(* Logix 5000 AddOnInstructionDefinition export; software revision 16.04 *)

ADD_ON_INSTRUCTION AMCI_ANG1E_Absolute_Move   (* revision 1.1, vendor AMCI *)
// Revision note:
// Version 1.1 added the slot_axis number and the input parameters can now be tags or discrete values.
VAR_INPUT
   slot_axis_number : INT; {required}
   Target_Position : DINT; {required}
   Programmed_Speed : DINT; {required}
   Acceleration : INT; {required}
   Deceleration : INT; {required}
END_VAR
VAR_IN_OUT
   AMCI_ANG1E_output_data : INT[10]; {required}
END_VAR
VAR
   Upper_Result_X_1000 : DINT;
   command_data_block : INT[10];
        [0]   // Command Bits MSW
        [1]   // Command Bits LSW
        [2]   // Upper Target Position
        [3]   // Lower Target Position
        [4]   // Upper Programmed Speed
        [5]   // Lower Programmed Speed
   index : INT;
END_VAR

ROUTINE Logic   (* ladder *)
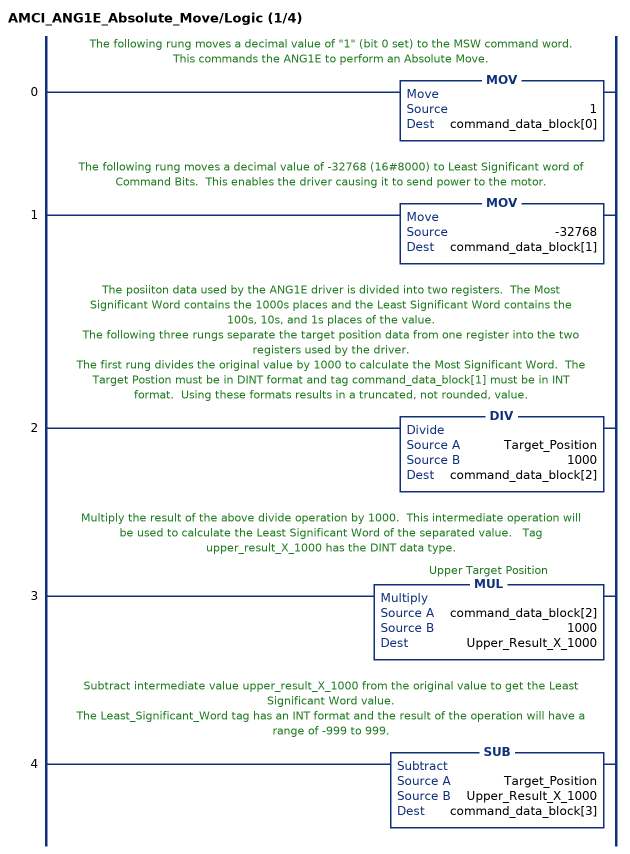
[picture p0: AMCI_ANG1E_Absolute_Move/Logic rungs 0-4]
   // The following rung moves a decimal value of "1" (bit 0 set) to the MSW command word.  This commands the ANG1E to perform an Absolute Move.
   0: MOV(1,command_data_block[0]);
   // The following rung moves a decimal value of -32768 (16#8000) to Least Significant word of Command Bits.  This enables the driver causing it to send power to the motor.
   1: MOV(-32768,command_data_block[1]);
   // The posiiton data used by the ANG1E driver is divided into two registers.  The Most Significant Word contains the 1000s places and the Least Significant Word contains the 100s, 10s, and 1s places of the value.
   // The following three rungs separate the target position data from one register into the two registers used by the driver.
   // The first rung divides the original value by 1000 to calculate the Most Significant Word.  The Target Postion must be in DINT format and tag command_data_block[1] must be in INT format.  Using these formats results in a truncated, not rounded, value.
   2: DIV(Target_Position,1000,command_data_block[2]);
   // Multiply the result of the above divide operation by 1000.  This intermediate operation will be used to calculate the Least Significant Word of the separated value.   Tag upper_result_X_1000 has the DINT data type.
   3: MUL(command_data_block[2],1000,Upper_Result_X_1000);
   // Subtract intermediate value upper_result_X_1000 from the original value to get the Least Significant Word value.
   // The Least_Significant_Word tag has an INT format and the result of the operation will have a range of -999 to 999.
   4: SUB(Target_Position,Upper_Result_X_1000,command_data_block[3]);
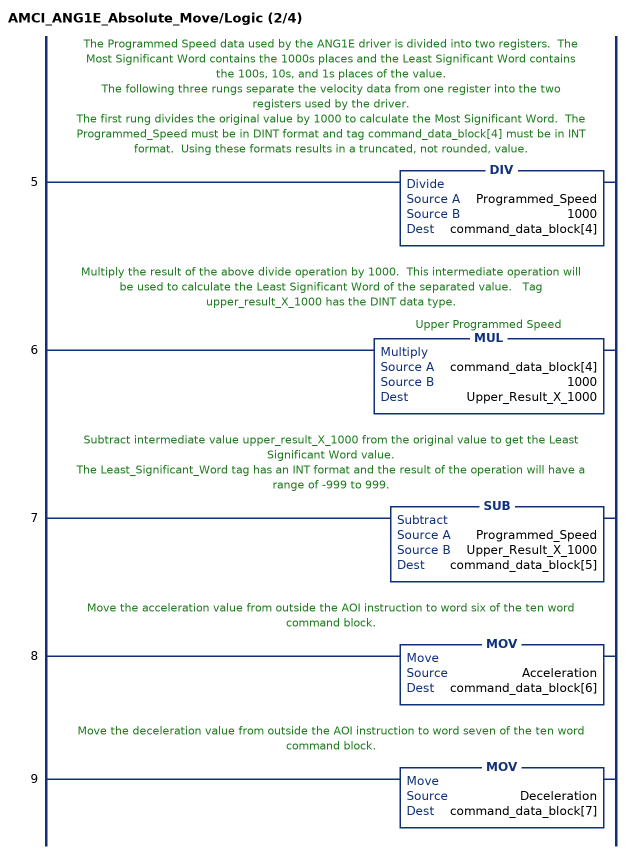
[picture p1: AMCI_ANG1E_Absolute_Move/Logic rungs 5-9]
   // The Programmed Speed data used by the ANG1E driver is divided into two registers.  The Most Significant Word contains the 1000s places and the Least Significant Word contains the 100s, 10s, and 1s places of the value.
   // The following three rungs separate the velocity data from one register into the two registers used by the driver.
   // The first rung divides the original value by 1000 to calculate the Most Significant Word.  The Programmed_Speed must be in DINT format and tag command_data_block[4] must be in INT format.  Using these formats results in a truncated, not rounded, value.
   5: DIV(Programmed_Speed,1000,command_data_block[4]);
   // Multiply the result of the above divide operation by 1000.  This intermediate operation will be used to calculate the Least Significant Word of the separated value.   Tag upper_result_X_1000 has the DINT data type.
   6: MUL(command_data_block[4],1000,Upper_Result_X_1000);
   // Subtract intermediate value upper_result_X_1000 from the original value to get the Least Significant Word value.
   // The Least_Significant_Word tag has an INT format and the result of the operation will have a range of -999 to 999.
   7: SUB(Programmed_Speed,Upper_Result_X_1000,command_data_block[5]);
   // Move the acceleration value from outside the AOI instruction to word six of the ten word command block.
   8: MOV(Acceleration,command_data_block[6]);
   // Move the deceleration value from outside the AOI instruction to word seven of the ten word command block.
   9: MOV(Deceleration,command_data_block[7]);
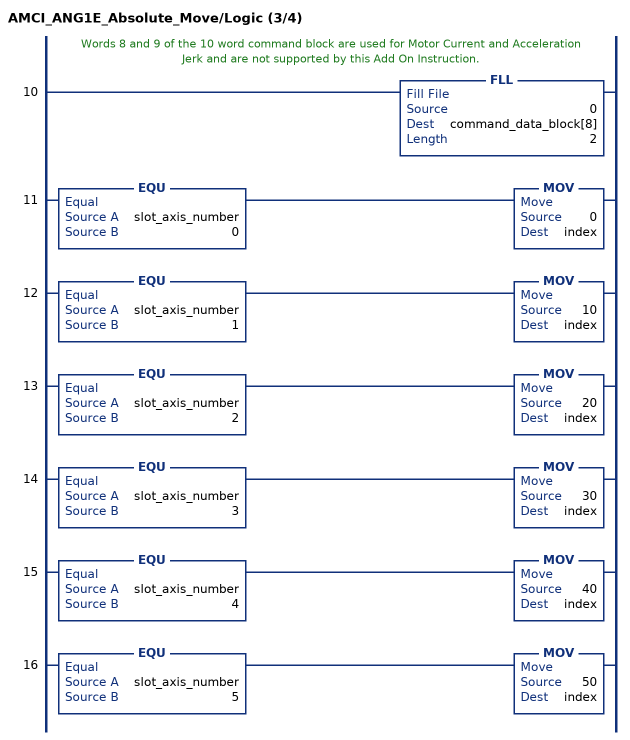
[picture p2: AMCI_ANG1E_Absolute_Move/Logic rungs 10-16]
   // Words 8 and 9 of the 10 word command block are used for Motor Current and Acceleration Jerk and are not supported by this Add On Instruction.
   10: FLL(0,command_data_block[8],2);
   11: EQU(slot_axis_number,0)MOV(0,index);
   12: EQU(slot_axis_number,1)MOV(10,index);
   13: EQU(slot_axis_number,2)MOV(20,index);
   14: EQU(slot_axis_number,3)MOV(30,index);
   15: EQU(slot_axis_number,4)MOV(40,index);
   16: EQU(slot_axis_number,5)MOV(50,index);
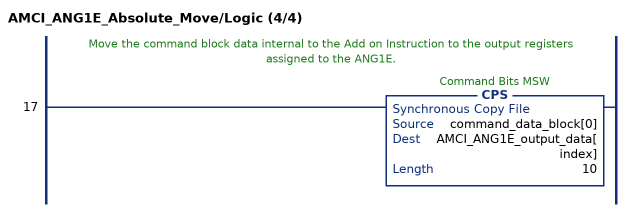
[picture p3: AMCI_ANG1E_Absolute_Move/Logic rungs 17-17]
   // Move the command block data internal to the Add on Instruction to the output registers assigned to the ANG1E.
   17: CPS(command_data_block[0],AMCI_ANG1E_output_data[index],10);
END_ROUTINE
END_ADD_ON_INSTRUCTION
